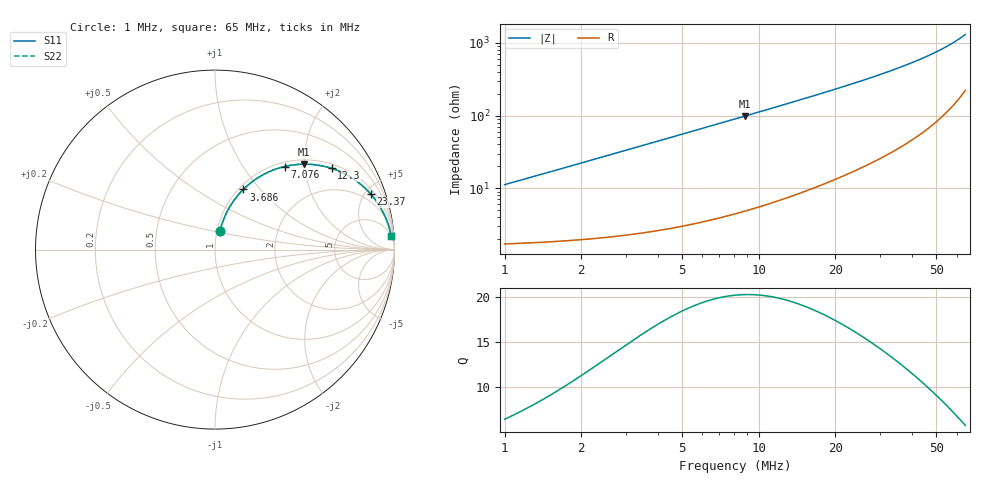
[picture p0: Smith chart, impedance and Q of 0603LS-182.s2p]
# MHz S MA R 50
!Freq  MagS11  AngS11  MagS21  AngS21  MagS12  AngS12  MagS22  AngS22
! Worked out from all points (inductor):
!   801 points, 1 MHz to 65 MHz, reference 50 ohm
!   read as one part in series: L = 1.76 uH near 1.021 MHz
!   highest Q = 20.3 at 8.856 MHz (marker M1), where L = 1.77 uH
!   S11 on the Smith chart (normalised r, x): 1 MHz: 1.03, +0.22; 3.686 MHz: 1.05, +0.82; 7.076 MHz: 1.08, +1.57; 12.3 MHz: 1.14, +2.76; 23.37 MHz: 1.34, +5.48; 65 MHz: 5, +26
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1  0.1094 75.0  0.9774 -6.2  0.9774 -6.2  0.1094 75.0
1.251538  0.1358 75.0  0.9737 -7.7  0.9737 -7.7  0.1358 75.0
1.49449  0.1612 74.5  0.9694 -9.2  0.9694 -9.2  0.1612 74.5
2.087017  0.2216 72.3  0.9564 -12.8  0.9564 -12.8  0.2216 72.3
2.809934  0.2917 69.0  0.9362 -16.9  0.9362 -16.9  0.2917 69.0
3.685831  0.3705 64.8  0.9065 -21.7  0.9065 -21.7  0.3705 64.8
4.401333  0.4293 61.4  0.8793 -25.4  0.8793 -25.4  0.4293 61.4
5.201167  0.4888 57.7  0.8467 -29.2  0.8467 -29.2  0.4888 57.7
7.076249  0.604 50.0  0.7674 -37.1  0.7674 -37.1  0.604 50.0
8.856196  0.6861 43.9  0.6946 -43.3  0.6946 -43.3  0.6861 43.9
11.67758  0.7765 36.3  0.5925 -50.9  0.5925 -50.9  0.7765 36.3
12.30309  0.7916 34.9  0.5725 -52.2  0.5725 -52.2  0.7916 34.9
14.38793  0.8329 30.7  0.512 -56.3  0.512 -56.3  0.8329 30.7
16.7385  0.8667 27.0  0.4543 -59.9  0.4543 -59.9  0.8667 27.0
19.37173  0.8938 23.6  0.4006 -63.2  0.4006 -63.2  0.8938 23.6
22.41922  0.9161 20.4  0.3498 -66.1  0.3498 -66.1  0.9161 20.4
23.37489  0.9216 19.6  0.3358 -66.9  0.3358 -66.9  0.9216 19.6
27.76721  0.9411 16.3  0.2813 -69.9  0.2813 -69.9  0.9411 16.3
33.15745  0.9562 13.3  0.2302 -72.5  0.2302 -72.5  0.9562 13.3
43.72065  0.9722 9.2  0.1601 -75.5  0.1601 -75.5  0.9722 9.2
54.43328  0.9802 6.3  0.1113 -76.6  0.1113 -76.6  0.9802 6.3
65  0.9844 4.3  0.07533 -75.9  0.07533 -75.9  0.9844 4.3
